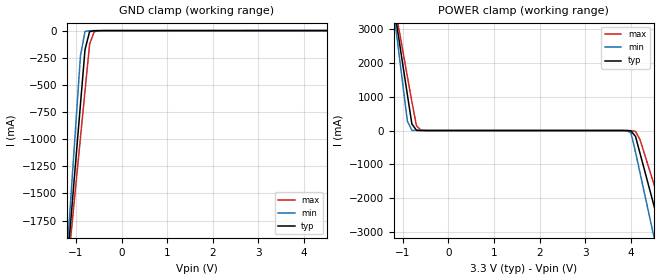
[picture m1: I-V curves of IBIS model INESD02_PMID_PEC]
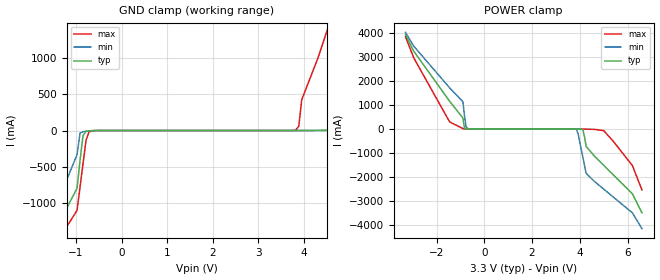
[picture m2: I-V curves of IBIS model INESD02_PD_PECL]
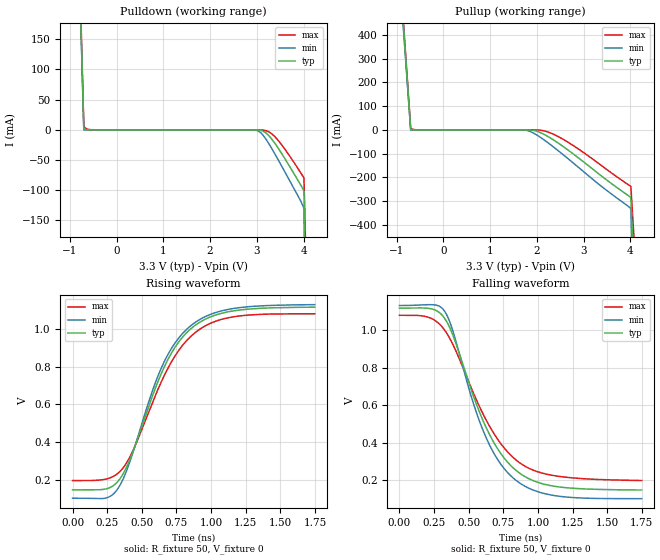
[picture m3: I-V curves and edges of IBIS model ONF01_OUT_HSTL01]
|   This file is an IBIS representation of the   |
|   Integrated Device Technology , Inc.   |
|   ICS852911I   |
|   Low Skew 1 to 9 LVHSTL Fanout Buffer   |
[IBIS Ver]   4.1
[File name]   852911i_3v3.ibs
[File Rev]   0.0
[Date]   2 Sep 2009 | Last modified
|   16 Dec 2004 | Generated
[Source]   Originated at Integrated Device Technology, Inc.
[Disclaimer]
IDT hereby grants the user of this IBIS model a non-exclusive,
nontransferable license to use this IBIS model under the following terms.
Before using this IBIS model, the user should read this license.
If the user does not accept these terms,  the IBIS model should be
returned to IDT within 30 days.
   The user is granted this license only to use the IBIS model and
is not granted rights to sell, load, rent, lease or license the IBIS
model in whole or in part, or in modified form to anyone other than
user. User may modify the IBIS model to suit its specific
applications but rights to derivative works and such modifications
shall belong to IDT.
   This IBIS model is provided on an "AS IS" basis and IDT makes
absolutely no warranty with respect to the information contained
herein. IDT DISCLAIMS AND CUSTOMER WAIVES ALL WARRANTIES, EXPRESS
OR IMPLIED, INCLUDING WARRANTIES OF MERCHANTABILITY OR FITNESS FOR
A PARTICULAR PURPOSE. The entire risk as to quality and performance
is with the Customer. ACCORDINGLY, IN NO EVENT SHALL THE COMPANY BE
LIABLE FOR ANY DAMAGES, WHETHER IN CONTRACT OR TORT,INCLUDING ANY
LOST PROFITS OR OTHER INCIDENTAL, CONSEQUENTIAL, EXEMPLARY, OR
PUNITIVE DAMAGES ARISING OUT OF THE USE OR APPLICATION OF THE IBIS
model provided in this package. Further, IDT reserves the right to
make changes without notice to any product herein to improve
reliability, function, or design. IDT does not convey any license
under patent rights or any other intellectual property rights,
including those of third parties.
   IDT is not obligated to provide maintenance or support
for the licensed IBIS model.
[Copyright]   Copyright 2004 by Integrated Device Technology , Inc.
[Component]   ICS852911i
[Manufacturer] Integrated Device Technology, Inc.
[Package]
|PLCC 28 Pin
|   typ   min   max
R_pkg   53.15m   49.2m   57.1m
L_pkg   3.123nH   2.878nH   3.368nH
C_pkg   0.65pF   0.632pF   0.667pF
[Pin] signal_name   model_name   R_pin   L_pin   C_pin
1   VDD   POWER   49.2m   2.878n   0.632p
2   nHSTL_CLK   INESD02_PMID_PEC   51.2m   3.038n   0.643p
3   PECL_CLK   INESD02_PD_PECL   53.8m   3.201n   0.655p
4   nPECL_CLK   INESD02_PMID_PEC   57.1m   3.368n   0.667p
5   nQ8   ONF01_OUT_HSTL01   57.1m   3.368n   0.667p
6   Q8   ONF01_OUT_HSTL01   53.8m   3.201n   0.655p
7   nQ7   ONF01_OUT_HSTL01   51.2m   3.038n   0.643p
8   VDDO   POWER   49.2m   2.878n   0.632p
9   Q7   ONF01_OUT_HSTL01   51.2m   3.038n   0.643p
10   nQ6   ONF01_OUT_HSTL01   53.8m   3.201n   0.655p
11   Q6   ONF01_OUT_HSTL01   57.1m   3.368n   0.667p
12   nQ5   ONF01_OUT_HSTL01   57.1m   3.368n   0.667p
13   Q5   ONF01_OUT_HSTL01   53.8m   3.201n   0.655p
14   nQ4   ONF01_OUT_HSTL01   51.2m   3.038n   0.643p
15   VDDO   POWER   49.2m   2.878n   0.632p
16   Q4   ONF01_OUT_HSTL01   51.2m   3.038n   0.643p
17   nQ3   ONF01_OUT_HSTL01   53.8m   3.201n   0.655p
18   Q3   ONF01_OUT_HSTL01   57.1m   3.368n   0.667p
19   nQ2   ONF01_OUT_HSTL01   57.1m   3.368n   0.667p
20   Q2   ONF01_OUT_HSTL01   53.8m   3.201n   0.655p
21   nQ1   ONF01_OUT_HSTL01   51.2m   3.038n   0.643p
22   VDDO   POWER   49.2m   2.878n   0.632p
23   Q1   ONF01_OUT_HSTL01   51.2m   3.038n   0.643p
24   nQ0   ONF01_OUT_HSTL01   53.8m   3.201n   0.655p
25   Q0   ONF01_OUT_HSTL01   57.1m   3.368n   0.667p
26   GND   GND   57.1m   3.368n   0.667p
27   CLK_SEL   INESD02_PD   53.8m   3.201n   0.655p
28   HSTL_CLK   INESD02_PD_PECL   51.2m   3.038n   0.643p
[Diff Pin]  inv_pin  vdiff tdelay_typ tdelay_min  tdelay_max
|Input
28   2   0.30 0  0  0
3   4   0.30 0  0  0
|Output
6   5   NA   0  0  0
9   7   NA   0  0  0
11   10   NA   0  0  0
13   12   NA   0  0  0
16   14   NA   0  0  0
18   17   NA   0  0  0
20   19   NA   0  0  0
23   21   NA   0  0  0
25   24   NA   0  0  0
| Models and submodels in the file (4): INESD02_PMID_PEC (Input), INESD02_PD_PECL (Input), ONF01_OUT_HSTL01 (Output_ECL), INESD02_PD (Input)
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[Model]   INESD02_PMID_PEC
Model_type   Input
Polarity   Non-Inverting
Vinl = 0.8V
Vinh = 2.0V
|   typ   min   max
C_comp   2pF   1.5pF   2.5pF
|   typ   min   max
[Voltage range]  3.3V   3.15V   3.45V
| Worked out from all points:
|   GND clamp passes 1 mA (typ) near -0.54 V on its own axis
|   POWER clamp passes 1 mA (typ) near -0.60 V on its own axis
[GND_clamp]
|Voltage   I(typ)   I(min)   I(max)
-3.3V     -12.83A    -15.14A    -11.37A
-1.2V     -2.195A    -2.092A    -2.281A
-1.1V     -1.689A    -1.472A    -1.849A
-900mV    -678.6mA   -232.7mA   -984.9mA
-800mV    -174mA     -7.255mA   -553.3mA
-700mV    -9.789mA   -1.13mA    -126.1mA
-600mV    -1.72mA    -254.4uA   -11.17mA
-500mV    -427uA     -99.72uA   -2.216mA
6.6V      76.52uA    70.16uA    79.2uA
[POWER_clamp]
|Voltage   I(typ)   I(min)   I(max)
-3.3V     22.38A     26.45A     19.82A
-1.2V     3.723A     3.545A     3.874A
-1.1V     2.836A     2.457A     3.116A
-900mV    1.063A     281mA      1.601A
-800mV    191.6mA    5.071mA    844mA
-600mV    678.1uA    76.63uA    10.7mA
3.9V      -1.629mA   -3.157mA   -831.1uA
4.1V      -173.9mA   -635.2mA   -23.94mA
4.5V      -2.195A    -3.116A    -1.568A
4.7V      -3.206A    -4.358A    -2.433A
4.9V      -4.218A    -5.6A      -3.298A
6.6V      -12.83A    -16.16A    -10.66A
[Model]   INESD02_PD_PECL
Model_type  Input
Polarity   Non-Inverting
Vinl = 0.8V
Vinh = 2.0V
|   typ   min   max
C_comp   2pF   1.5pF   2.5pF
|   typ   min   max
[Voltage range]  3.3V   3.15V   3.45V
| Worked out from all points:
|   GND clamp passes 1 mA (typ) near -0.59 V on its own axis
|   POWER clamp passes 1 mA (typ) near -0.70 V on its own axis
[GND_clamp]
-3.3V     -3.894A    -4.294A    -3.674A
-1.6V     -1.569A    -1.322A    -1.74A
-974.8mV  -794.1mA   -331.5mA   -1.096A
-843.4mV  -68.33mA   -15.34mA   -452.9mA
-646.5mV  -1.912mA   -4.151mA   -2.665mA
3.818V    89.38uA    70.49uA    7.198mA
3.95V     342.2uA    75.94uA    423.8mA
4.6V      7.437mA    165.5uA    1.553A
4.9V      78.32mA    440.9uA    2.118A
5.5V      1.293A     2.769mA    3.249A
6.25V     2.651A     112.4mA    4.38A
6.6V      3.331A     896.1mA    4.946A
[POWER_clamp]
-3.3V     3.923A     4.017A     3.838A
-2.95V    3.23A      3.44A      2.951A
-1.45V    1.149A     1.709A     289.6mA
-896.9mV  456.5mA    1.133A     15.4mA
-762.9mV  4.223mA    91.07mA    1.486mA
-695.9mV  792.2uA    10.73mA    555.6uA
3.861V    -556.7uA   -26.14mA   -39.45uA
4.129V    -41.85mA   -1.19A     -4.904mA
4.263V    -724.2mA   -1.847A    -12.04mA
5V        -1.514A    -2.505A    -71.38mA
6.2V      -2.701A    -3.492A    -1.525A
6.6V      -3.492A    -4.151A    -2.536A
[Model]   ONF01_OUT_HSTL01
Model_type   Output_ECL
Polarity   Non-Inverting
|   typ   min   max
C_comp   2pF   1.5pF   2.5pF
Vmeas = 0.600V
Rref = 50
Cref = 0
Vref = 0V
|   typ   min   max
[Voltage range]   3.3V   3.135V   3.465V
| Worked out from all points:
|   rising waveform, R_fixture 50, V_fixture 0: 20-80 % time 326ps typ, 318ps min, 337ps max; typ from 0.145 V to 1.12 V
|   falling waveform, R_fixture 50, V_fixture 0: 20-80 % time 321ps typ, 298ps min, 354ps max; typ from 1.12 V to 0.147 V
[Pulldown]
|Voltage   I (typ)   I (min)   I (max)
-3.3V     9.786A     12.03A     8.45A
-1.22V    1.462A     1.413A     1.509A
-700mV    628.3uA    69.5uA     5.973mA
-474.4mV  5.149uA    100.6nA    52.71uA
2.868V    -2.24uA    -24.76uA   -402.6nA
3.084V    -841uA     -4.706mA   -151.9uA
3.245V    -8.501mA   -21.25mA   -2.833mA
3.407V    -24.43mA   -42.5mA    -12.93mA
3.838V    -78.03mA   -103.2mA   -58.94mA
4.01V     -100.9mA   -130.6mA   -79.6mA
4.528V    -2.529A    -3.788A    -1.727A
6.6V      -15.7A     -20.59A    -12.71A
[Pullup]
|Voltage   I (typ)   I (min)   I (max)
-3.3V     9.786A     12.03A     8.45A
-1.22V    1.462A     1.413A     1.509A
-700mV    628.3uA    69.5uA     5.973mA
-528.3mV  18.79uA    633.1nA    153.9uA
1.736V    -34.65uA   -846.1uA   -282.1nA
1.951V    -3.39mA    -16.38mA   -140.8uA
2.221V    -26.41mA   -52.03mA   -8.076mA
2.437V    -53.07mA   -84.82mA   -26.45mA
2.76V     -98.86mA   -136.7mA   -63.97mA
4.01V     -284.5mA   -332.4mA   -238.3mA
4.528V    -2.712A    -3.986A    -1.887A
6.6V      -15.7A     -20.55A    -12.73A
[Ramp]
|   typ   min   max
dV/dt_r   0.776/0.51n   0.824/0.504n   0.708/0.52n
dV/dt_f   0.776/0.496n   0.827/0.462n   0.704/0.545n
R_load =   50.0000
[Rising Waveform]
R_fixture = 50
V_fixture = 0
V_fixture_max = 0
V_fixture_min = 0
C_fixture = 0.0p
| Time   typ   min   max
0s        145.3mV    100.9mV    194.4mV
234.7ps   149.3mV    101mV      201.6mV
325.8ps   188.8mV    150.4mV    232.2mV
430.9ps   338.8mV    332.5mV    345.7mV
564.1ps   618.8mV    644.8mV    586.1mV
644.6ps   770.4mV    799.4mV    725.8mV
744.5ps   908.2mV    930.6mV    862.2mV
854.9ps   1.002V     1.018V     961.4mV
1.144ns   1.094V     1.107V     1.062V
1.748ns   1.116V     1.129V     1.081V
[Falling Waveform]
R_fixture = 50
V_fixture = 0
V_fixture_max = 0
V_fixture_min = 0
C_fixture = 0.0p
| Time   typ   min   max
0s        1.116V     1.13V      1.078V
210.2ps   1.115V     1.135V     1.067V
327.6ps   1.061V     1.098V     997.8mV
381.9ps   980.2mV    1.004V     928.8mV
520.3ps   676.6mV    640.9mV    687.8mV
611.4ps   503.5mV    450.8mV    540.8mV
718.2ps   356.1mV    299.1mV    407.8mV
837.3ps   254.6mV    201.1mV    309.8mV
1.116ns   167.5mV    117.9mV    223.9mV
1.748ns   147.2mV    101.1mV    197.9mV
